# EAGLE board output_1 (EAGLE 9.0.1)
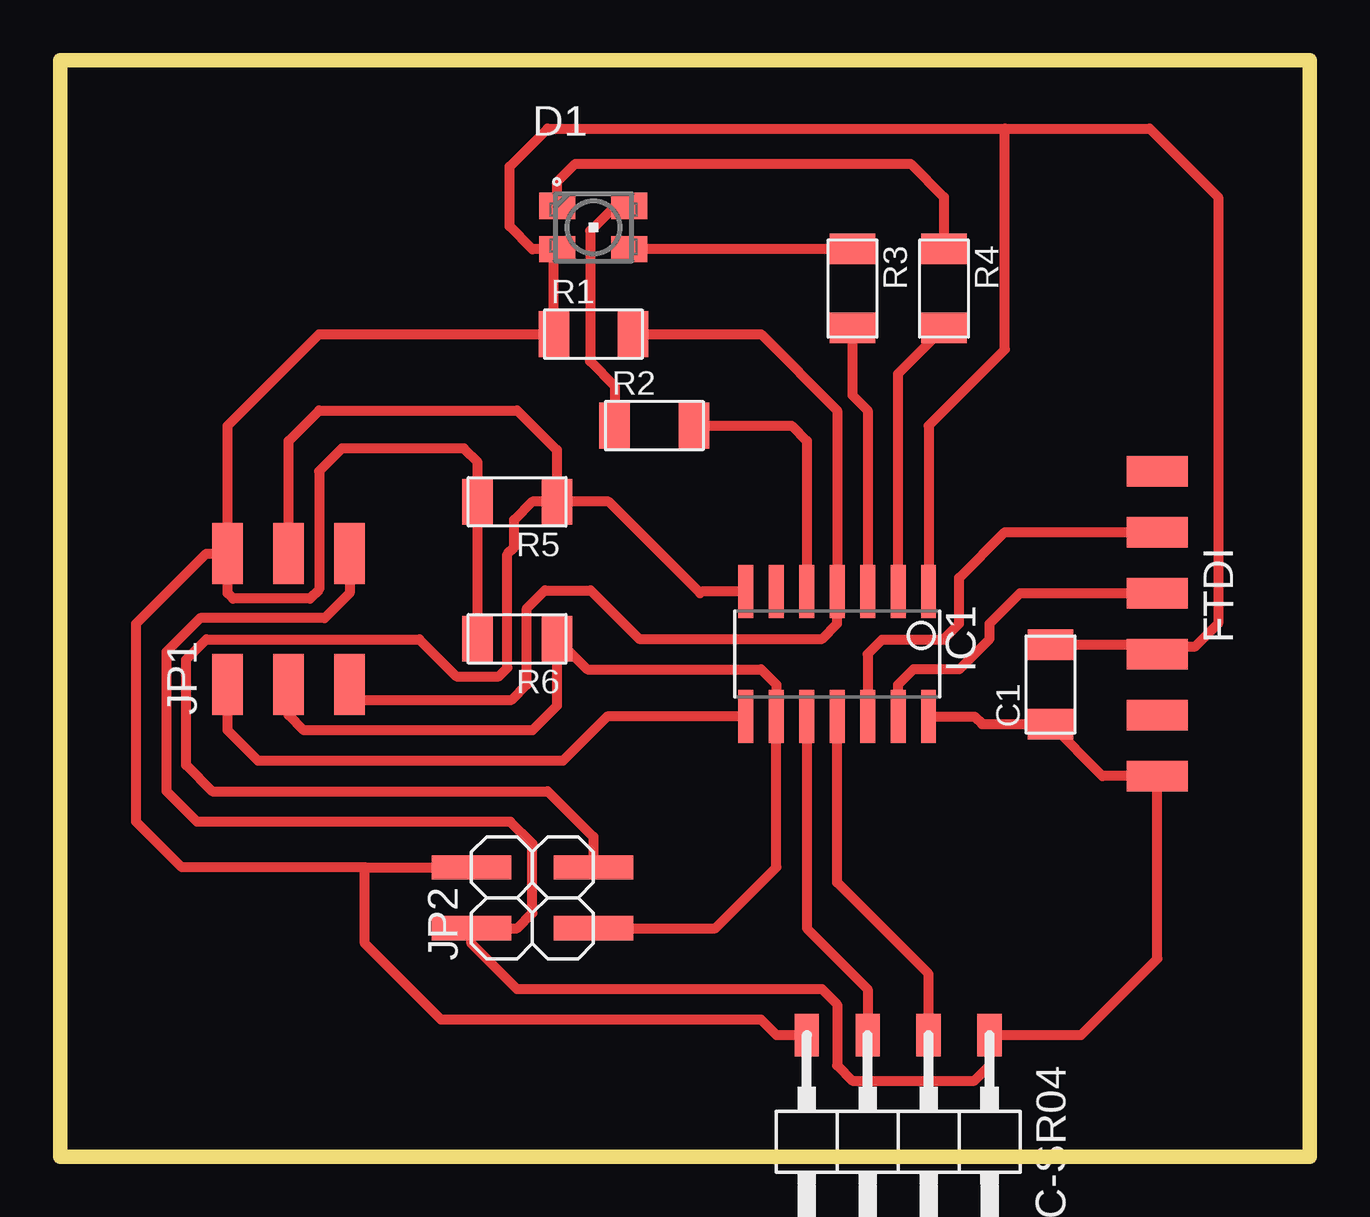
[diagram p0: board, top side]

Size 52.07 x 45.72 mm. Coordinates in mm from the lower left corner, seen from the top.
Outline: 0,45.72 52.07,45.72 52.07,0 0,0 0,45.72
Copper layers (1*16): Top 0.035mm / dielectric 1.5mm / Bottom 0.035mm
Design rules "ReglasDeDiseño": minimum track width 16mil, minimum drill 0.35mm, track to track 16mil, track to pad 16mil, pad to pad 16mil, via to via 16mil, smd to smd 6mil, copper to edge 40mil, drill to drill 16mil, minimum pad ring 10mil, minimum via ring 8mil, stop-mask expansion 4mil, vias tented up to drill 0mil, thermal gap 10mil

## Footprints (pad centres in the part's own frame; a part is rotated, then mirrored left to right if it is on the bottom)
C1206FAB = smd 1.27 x 1.905: 1 -1.651,0; 2 1.651,0
P-LCC-4 = smd 1.1 x 1.5: A 0.902,-1.5; B 0.902,1.5; G -0.902,1.5; R -0.902,-1.5
1X06SMD = smd 2.54 x 1.27: 1 0,6.35; 2 0,3.81; 3 0,1.27; 4 0,-1.27; 5 0,-3.81; 6 0,-6.35
1X04SMD/90 = smd 1.016 x 1.778: 1 -1.27,-5.08; 2 1.27,-5.08; 3 3.81,-5.08; 4 6.35,-5.08
SOIC14 = smd 0.61 x 2.21: 1 -3.81,-2.603; 2 -2.54,-2.603; 3 -1.27,-2.603; 4 0,-2.603; 5 1.27,-2.603; 6 2.54,-2.603; 7 3.81,-2.603; 8 3.81,2.603; 9 2.54,2.603; 10 1.27,2.603; 11 0,2.603; 12 -1.27,2.603; 13 -2.54,2.603; 14 -3.81,2.603
2X03SMD = smd 2.54 x 1.27: 1 -2.54,2.54; 2 2.92,2.54; 3 -2.54,0; 4 2.92,0; 5 -2.54,-2.54; 6 2.92,-2.54
2X02SMD = smd 1.016 x 3.302: 1 -1.27,-3.81; 2 -1.27,1.27; 3 1.27,-3.81; 4 1.27,1.27
R1206FAB = smd 1.27 x 1.905: 1 -1.651,0; 2 1.651,0

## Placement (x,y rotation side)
C1  1uF  [C1206FAB]  41.27,19.69 90 top
D1  LEDRGBNEW  [P-LCC-4]  22.22,38.73 270 top
FTDI  FTDI-SMD-HEADER  [1X06SMD]  45.72,22.23 180 top
HC-SR04  [1X04SMD/90]  37.47,0 180 top
IC1  ATTINY44-SSU  [SOIC14]  32.38,20.95 180 top
JP1  AVRISPSMD  [2X03SMD]  9.52,22.23 90 top
JP2  [2X02SMD]  18.41,10.79 90 top
R1  10k  [R1206FAB]  22.22,34.29 0 top
R2  499  [R1206FAB]  24.77,30.48 0 top
R3  499  [R1206FAB]  33.02,36.2 270 top
R4  499  [R1206FAB]  36.83,36.2 270 top
R5  10k  [R1206FAB]  19.05,27.3 180 top
R6  10k  [R1206FAB]  19.05,21.59 180 top

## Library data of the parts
C1 D1 FTDI IC1 JP1 R1-R6 = fab
HC-SR04 JP2 = pinhead-1

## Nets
ECHO: HC-SR04.2 IC1.11
GND: C1.1 FTDI.1 HC-SR04.1 IC1.14 JP1.6 JP2.2
MISO: IC1.8 JP1.1
N$1: D1.R R4.1
N$2: FTDI.2
N$4: D1.B R3.1
N$5: D1.G R2.1
N$6: FTDI.6
N$13: IC1.6
PB0: IC1.2 R4.2
PB1: IC1.3 R3.2
PB2: IC1.5 R2.2
RST: IC1.4 JP1.5 R1.2
RX: FTDI.5 IC1.12
SCL: IC1.9 JP1.3 JP2.1 R6.1
SDA: IC1.7 JP1.4 JP2.3 R5.1
TRG: HC-SR04.3 IC1.10
TX: FTDI.4 IC1.13
VCC: C1.2 D1.A FTDI.3 HC-SR04.4 IC1.1 JP1.2 JP2.4 R1.1 R5.2 R6.2

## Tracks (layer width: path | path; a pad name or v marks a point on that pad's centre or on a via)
ECHO
  Top 0.406: HC-SR04.2 36.2,7.62 32.38,11.43 IC1.11
GND
  Top 0.406: IC1.14 38.1,18.35 38.42,18.03 C1.1 43.43,15.88 FTDI.1 45.72,8.25 42.55,5.08 HC-SR04.1 38.73,3.81 38.1,3.17 33.02,3.17 32.38,3.81 32.38,6.35 31.75,6.98 19.05,6.98 17.14,8.89 JP2.2 19.05,9.53 19.68,10.16 19.68,13.06 18.77,13.97 5.71,13.97 4.44,15.24 4.44,21.06 5.84,22.45 11.02,22.45 12.06,23.5 JP1.6
MISO
  Top 0.406: JP1.1 6.98,17.78 8.25,16.51 20.95,16.51 22.8,18.35 IC1.8
N$1
  Top 0.406: D1.R 20.72,40.64 21.47,41.39 35.45,41.39 36.83,40 R4.1
N$4
  Top 0.406: R3.1 33.01,37.83 D1.B
N$5
  Top 0.406: D1.G 23.13,39.64 22.09,38.59 22.09,33.16 23.11,32.13 R2.1
PB0
  Top 0.406: IC1.2 34.92,32.64 R4.2
PB1
  Top 0.406: R3.2 33.02,31.75 33.66,31.11 IC1.3
PB2
  Top 0.406: IC1.5 31.11,29.84 30.48,30.48 R2.2
RST
  Top 0.406: R1.2 29.21,34.29 32.38,31.11 IC1.4 32.38,22.23 31.75,21.59 24.13,21.59 22.11,23.61 20.21,23.61 19.46,22.86 19.46,19.69 18.82,19.05 12.06,19.05 JP1.5
RX
  Top 0.406: IC1.12 33.66,20.95 34.26,21.56 36.86,21.56 36.86,21.62 37.47,22.23 37.47,24.13 39.37,26.04 FTDI.5
SCL
  Top 0.406: JP1.3 9.52,18.41 10.16,17.78 19.68,17.78 20.7,18.8 R6.1 21.97,20.32 29.21,20.32 29.84,19.69 IC1.9 29.84,12.06 27.3,9.53 JP2.1
SDA
  Top 0.406: IC1.7 26.73,23.56 26.67,23.5 22.86,27.3 R5.1 | JP1.4 9.52,29.84 10.79,31.11 19.05,31.11 20.7,29.46 R5.1 | JP2.3 22.22,13.34 20.32,15.24 6.35,15.24 5.26,16.33 5.26,20.73 6.1,21.56 14.97,21.56 16.51,20.03 18.29,20.03 18.64,20.38 18.64,25.12 18.92,25.4 18.92,26.54 19.68,27.3 R5.1
TRG
  Top 0.406: HC-SR04.3 33.66,6.98 31.11,9.53 IC1.10
TX
  Top 0.406: IC1.13 34.92,19.69 35.56,20.32 37.47,20.32 38.73,21.59 38.73,22.23 40,23.5 FTDI.4
VCC
  Top 0.406: C1.2 45.34,21.34 FTDI.3 46.04,21.27 47.31,21.27 48.26,22.23 48.26,40 45.4,42.86 39.37,42.86 | 12.7,12.06 12.7,8.89 15.88,5.71 29.21,5.71 29.84,5.08 HC-SR04.4 | 12.7,12.06 JP2.4 | D1.A 20.32,37.83 | 20.32,37.83 19.68,37.83 18.73,38.79 18.73,41.28 20.32,42.86 39.37,42.86 | IC1.1 36.2,30.48 39.37,33.66 39.37,42.86 | 20.32,37.83 20.57,37.58 R1.1 10.79,34.29 6.98,30.48 JP1.2 | JP1.2 6.98,23.5 7.21,23.27 10.41,23.27 10.79,23.65 10.79,28.57 11.75,29.53 16.83,29.53 17.4,28.96 R5.2 R6.2 | 12.7,12.06 5.08,12.06 3.17,13.97 3.17,22.23 6.09,25.14 JP1.2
